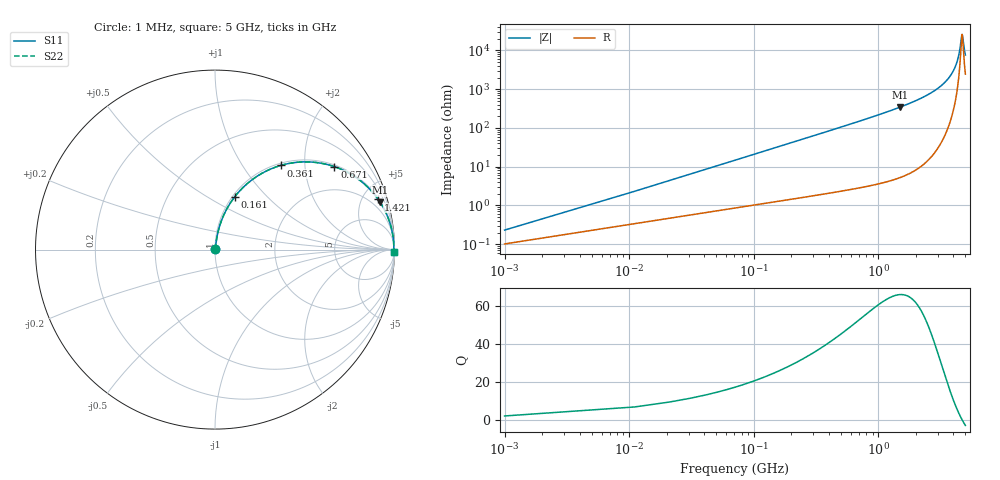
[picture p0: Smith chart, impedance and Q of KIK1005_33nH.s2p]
!version-3
!date-01.2023
!Series
# MHz S RI R 50
!Freq ReS11 ImS11 ReS21 ImS21 ReS12 ImS12 ReS22 ImS22
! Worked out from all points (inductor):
!   501 points, 1 MHz to 5 GHz, reference 50 ohm
!   read as one part in series: L = 33 nH near 21 MHz
!   highest Q = 66 at 1.501 GHz (marker M1), where L = 36.7 nH
!   self-resonance near 4.701 GHz
!   S11 on the Smith chart (normalised r, x): 1 MHz: 1.00, +0.00; 161 MHz: 1.03, +0.67; 361 MHz: 1.04, +1.51; 671 MHz: 1.05, +2.84; 1.421 GHz: 1.10, +6.48; 5 GHz: open
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1  0.00102 0.00207  0.999 -0.00207  0.999 -0.00207  0.00102 0.00207
31  0.00966 0.0633  0.9903 -0.0633  0.9903 -0.0633  0.00966 0.0633
41  0.0135 0.0833  0.9865 -0.0833  0.9865 -0.0833  0.0135 0.0833
61  0.0232 0.1226  0.9768 -0.1226  0.9768 -0.1226  0.0232 0.1226
91  0.043 0.1789  0.957 -0.1789  0.957 -0.1789  0.043 0.1789
161  0.1097 0.2938  0.8903 -0.2938  0.8903 -0.2938  0.1097 0.2938
251  0.2213 0.3999  0.7787 -0.3999  0.7787 -0.3999  0.2213 0.3999
361  0.3653 0.4687  0.6347 -0.4687  0.6347 -0.4687  0.3653 0.4687
671  0.6656 0.4622  0.3344 -0.4622  0.3344 -0.4622  0.6656 0.4622
841  0.7606 0.418  0.2394 -0.418  0.2394 -0.418  0.7606 0.418
1421  0.9096 0.2792  0.0904 -0.2792  0.0904 -0.2792  0.9096 0.2792
1501  0.9197 0.2642  0.0803 -0.2642  0.0803 -0.2642  0.9197 0.2642
1671  0.937 0.2354  0.063 -0.2354  0.063 -0.2354  0.937 0.2354
2501  0.9786 0.135  0.0214 -0.135  0.0214 -0.135  0.9786 0.135
3341  0.9922 0.0708  0.00785 -0.0708  0.00785 -0.0708  0.9922 0.0708
3821  0.9951 0.0427  0.00488 -0.0427  0.00488 -0.0427  0.9951 0.0427
4171  0.9961 0.0246  0.00393 -0.0246  0.00393 -0.0246  0.9961 0.0246
4441  0.9963 0.0118  0.00371 -0.0118  0.00371 -0.0118  0.9963 0.0118
4701  0.9962 0.000245  0.00384 -0.000245  0.00384 -0.000245  0.9962 0.000245
4741  0.9961 -0.00148  0.00389 0.00148  0.00389 0.00148  0.9961 -0.00148
4891  0.9959 -0.0078  0.00411 0.0078  0.00411 0.0078  0.9959 -0.0078
5000  0.9957 -0.0123  0.00433 0.0123  0.00433 0.0123  0.9957 -0.0123
